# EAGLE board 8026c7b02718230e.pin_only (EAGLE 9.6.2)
REV: A

Size 10.16 x 17.14 mm. Coordinates in mm from the lower left corner, seen from the top.
Outline: 0,0 0,14.61 arc-90 2.54,17.14 7.62,17.14 arc-90 10.16,14.61 10.16,0 0,0
Copper layers (1*16): Top 0.035mm / dielectric 1.5mm / Bottom 0.035mm
Design rules "adafruit *": minimum track width 8mil, minimum drill 15.5mil, track to track 8mil, track to pad 8mil, pad to pad 8mil, via to via 8mil, smd to smd 8mil, copper to edge 10mil, drill to drill 8mil, minimum pad ring 10mil, minimum via ring 8mil, stop-mask expansion 2mil, vias tented up to drill 20mil, thermal gap 10mil

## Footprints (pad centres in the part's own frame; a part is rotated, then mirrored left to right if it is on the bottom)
0805-NO = smd 1.24 x 1.5: 1 -0.95,0; 2 0.95,0
FIDUCIAL_1MM = smd 1 x 1: 1 0,0
MPM3610 = smd 0.7 x 0.25: 1 -1.45,1.55; 4 -1.45,-0.4; 5 -1.45,-1.25; 6 -1.45,-2.1; 7 1.45,-2.1; 8 1.45,-1.25; 9 1.45,-0.4; 12 1.45,1.55 | smd 1.1 x 0.25: 2 -1.25,0.9; 3 -1.25,0.25; 10 1.25,0.25; 11 1.25,0.9 | smd 0.25 x 0.7: 13 1.25,2.45; 14 0.75,2.45; 17 -0.75,2.45; 18 -1.25,2.45 | smd 0.25 x 1.1: 15 0.25,2.25; 16 -0.25,2.25
1X04_ROUND = drill 1 pad 1.778: 1 -3.81,0; 2 -1.27,0; 3 1.27,0; 4 3.81,0
0603-NO = smd 1.075 x 1: 1 -0.85,0; 2 0.85,0
MOUNTINGHOLE_2.5_PLATED = drill 2.5 pad 3.2: P$1 0,0

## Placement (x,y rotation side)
C1  22uF  [0805-NO]  3.43,4.83 0 top
C2  22uF  [0805-NO]  7.24,6.35 270 top
FID1  FIDUCIAL_1MM  [FIDUCIAL_1MM]  1.78,15.62 0 top
IC1  MPM3610  [MPM3610]  3.43,7.62 270 top
JP1  [1X04_ROUND]  5.08,2.54 180 top
R1  75K  [0603-NO]  7.87,8.76 180 top
R2  75K  [0603-NO]  6.86,10.79 180 top
R3  24K  [0603-NO]  3.81,10.79 180 top
U$9  MOUNTINGHOLE2.5  [MOUNTINGHOLE_2.5_PLATED]  5.08,14.61 0 top
U$10  [PCBFEAT-REV-040]  1.78,14.61 0 bottom
U$11  [ADAFRUIT_2.5MM]  2.79,11.3 90 top

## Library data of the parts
C1 C2 IC1 JP1 R1-R3 U$11 = microbuilder
FID1 U$9 = microbuilder; BOM: EXCLUDE
U$10 = microbuilder; REV: A

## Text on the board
tPlace: MPM / 3610 | GND | 3V | Vin | En
bPlace: Vin: 4.5-21V / Vout:3.3V / 1.2A Max | MPM3610

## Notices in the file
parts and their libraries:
microbuilder: This work is placed in the public domain, and may be freely used for commercial and non-commercial work with the following conditions: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
